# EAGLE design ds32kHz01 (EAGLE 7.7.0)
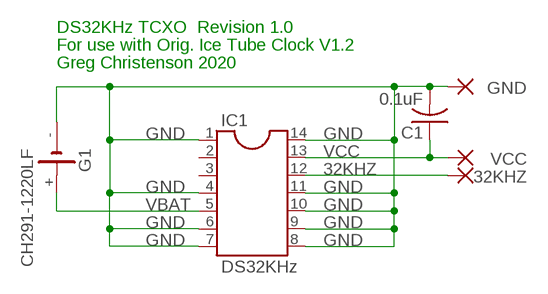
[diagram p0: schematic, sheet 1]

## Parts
32KHZ  WIREPAD1,6/0,9  [1,6/0,9]
C1  0.1uF  C-US025-025X050  [C025-025X050]
G1  CH291-1220LF  [CH291-1220LF]
GND  WIREPAD1,6/0,9  [1,6/0,9]
IC1  DS32KHz  DIL14S  [SOCKET-14]
VCC  WIREPAD1,6/0,9  [1,6/0,9]

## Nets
32KHZ: 32KHZ.1(P) IC1.12
GND: C1.2 G1.- GND.1(P) IC1.1 IC1.4 IC1.6 IC1.7 IC1.8 IC1.9 IC1.10 IC1.11 IC1.14
VBAT: G1.+ IC1.5
VCC: C1.1 IC1.13 VCC.1(P)
Unconnected: IC1.2 IC1.3

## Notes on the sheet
- DS32KHz TCXO  Revision 1.0
- For use with Orig. Ice Tube Clock V1.2
- Greg Christenson 2020

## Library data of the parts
32KHZ GND VCC = wirepad:WIREPAD: Wire PAD connect wire on PCB
C1 = resistor:C-US: CAPACITOR, American symbol
G1 = battery:CH291-1220LF: Battery Holder, SMT, 12mm
IC1 = ic-package:DIL14: Dual In Line / Socket

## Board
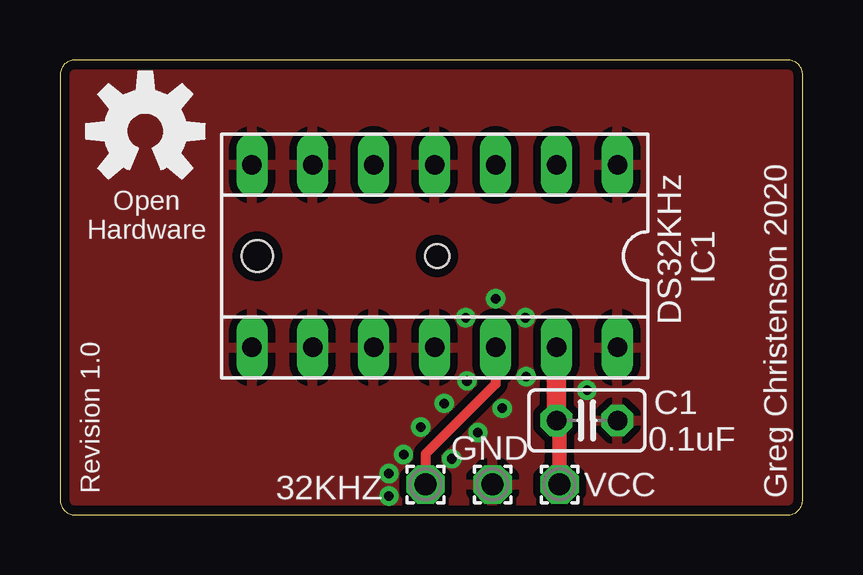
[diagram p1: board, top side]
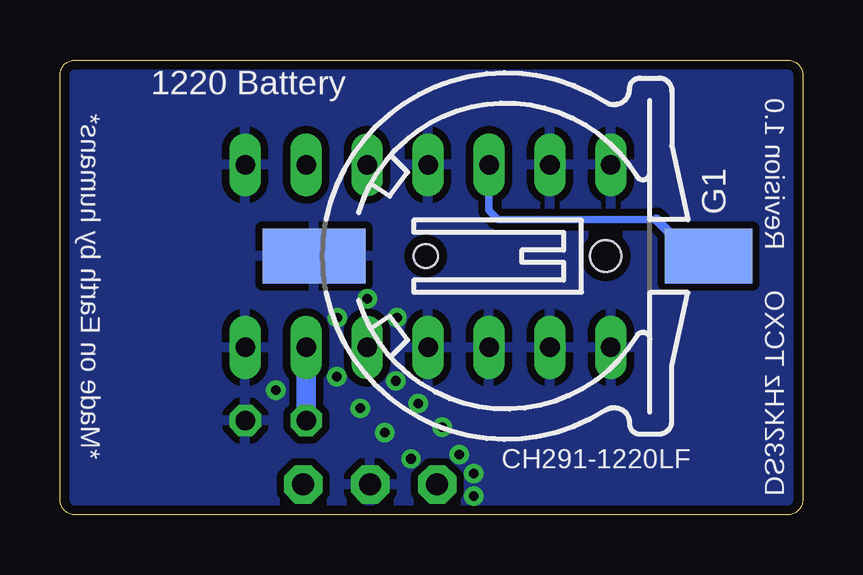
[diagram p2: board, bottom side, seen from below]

Size 30.97 x 18.97 mm. Coordinates in mm from the lower left corner, seen from the top.
Outline: 0,18.34 0,0.64 arc90 0.64,0 30.33,0 arc90 30.97,0.64 30.97,18.34 arc90 30.33,18.97 0.64,18.97 arc90 0,18.34
Copper layers (1*16): Top 0.035mm / dielectric 1.5mm / Bottom 0.035mm
Design rules "default *": minimum track width 10mil, minimum drill 24mil, track to track 12mil, track to pad 12mil, pad to pad 12mil, via to via 12mil, smd to smd 8mil, copper to edge 15mil, drill to drill 8mil, minimum pad ring 10mil, minimum via ring 8mil, stop-mask expansion 4mil, vias tented up to drill 20mil, thermal gap 12mil

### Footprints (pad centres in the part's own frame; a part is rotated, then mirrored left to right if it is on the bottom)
1,6/0,9 = drill 0.914 pad 1.6 octagon: 1 0,0
C025-025X050 = drill 0.813 octagon: 1 -1.27,0; 2 1.27,0
CH291-1220LF = smd 2.3 x 3.66: + 0,-2.296 | smd 2.3 x 4.3: - 0,14.146 | hole 1.3: 0,2 | hole 1: 0,9.5
SOCKET-14 = drill 0.813 long: 1 -7.62,-3.81; 2 -5.08,-3.81; 3 -2.54,-3.81; 4 0,-3.81; 5 2.54,-3.81; 6 5.08,-3.81; 7 7.62,-3.81; 8 7.62,3.81; 9 5.08,3.81; 10 2.54,3.81; 11 0,3.81; 12 -2.54,3.81; 13 -5.08,3.81; 14 -7.62,3.81

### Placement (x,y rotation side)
32KHZ  15.24,1.27 0 top
C1  21.97,3.94 0 top
G1  6.22,10.79 90 bottom
GND  18.03,1.27 0 top
IC1  15.62,10.79 180 top
U$1  [OSHW-LOGO-M]  3.56,16 0 top
VCC  20.83,1.27 0 top

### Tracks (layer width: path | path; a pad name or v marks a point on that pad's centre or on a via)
32KHZ
  Top 0.406: IC1.12 18.16,5.46 15.24,2.54 32KHZ.1
GND  (via drill 0.4)
  other vias: 14.33,2.51 13.72,0.79 16.33,2.34 15.04,3.66 16.03,4.65 17.42,3.43 18.44,4.45 19.43,5.77 19.41,8.23 18.16,9.02 16.92,8.23 16.97,5.59 13.72,1.73 21.97,5.21
  pour Top: 0,0 30.99,0 30.99,18.92 0,18.92
  pour Bottom: 0,0 30.99,0 30.99,18.92 0,18.92
VBAT
  Bottom 0.305: IC1.5 13.08,12.7 12.7,12.32 6.1,12.32
  Bottom 0.406: 6.1,12.32 4.57,10.79 G1.+
VCC
  Top 0.61: VCC.1 20.83,3.81 C1.1
  Top 0.813: IC1.13 C1.1
  Bottom 0.813: IC1.13 C1.1

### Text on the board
tNames: Open / Hardware | Revision 1.0 | Greg Christenson 2020
bNames: 1220 Battery | Revision 1.0 | *Made on Earth by humans* | DS32KHz TCXO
